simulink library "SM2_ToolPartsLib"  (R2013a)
settings: Solver=ode45  StartTime=0.0  StopTime=10.0  RelTol=1e-3
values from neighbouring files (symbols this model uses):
  m = v*BEAM.rho    [FlexBeamModelConstruct2.m]    (also in FlexBeamModelConstruct3.m = BEAM.rho*v; FlexBeam_1D_Construct.m = REF.m/REF.l*a.*(linspace(1-OPT.MassBiais+1e-6,1+OPT.MassBiai; FlexBeam_3D_Construct.m = REF.m/REF.l*a.*(linspace(1-OPT.MassBiais+1e-6,1+OPT.MassBiai; FreeFlexBeam_3D_Construct.m = REF.m/REF.l*a.*tmp2)
  N = D(1)+(H4^2+H3^2)/H2^2-(E(1)*H4+F(1)*H3)/H2    [MGD.m]    (also in MGD2.m)
  s = -sign(imag(KGZ_fr_tmp))    [LinprogReguliOptimFunc_1.m]    (also in LinprogReguliOptimFunc_2.m; LinprogReguliOptimFunc_1 - Copie.m)
  X = cos(phi(i))*x+sin(phi(i))*y    [MGI.m]
  Y = fft(y(:,i),NFFT)/L    [fft_bis.m]    (also in MGI.m = -sin(phi(i))*x+cos(phi(i))*y)
  Z = z    [MGI.m]
undefined symbols (not defined in the file or in its folder): deg, kg, SimParam
libraries: sm_lib x12, nesl_utility x1

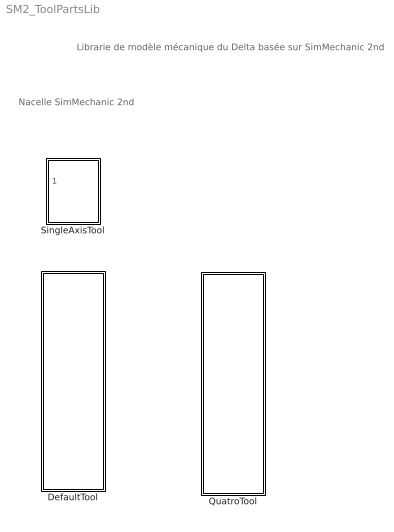
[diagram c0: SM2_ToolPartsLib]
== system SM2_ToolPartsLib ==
  note: Librarie de modèle mécanique du Delta basée sur SimMechanic 2nd
  note: Nacelle SimMechanic 2nd
  DefaultTool : Subsystem  InitFcn=SimParam.Tool = Tool_paramInitFnc(RawParam);
  QuatroTool : Subsystem  InitFcn=SimParam.Tool = Tool_paramInitFnc(RawParam);
  SingleAxisTool : Subsystem  InitFcn=SimParam.Tool = Tool_paramInitFnc(RawParam);

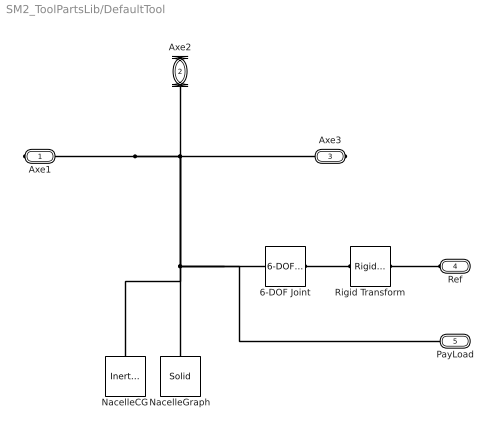
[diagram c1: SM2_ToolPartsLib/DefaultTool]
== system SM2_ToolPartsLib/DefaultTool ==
  6-DOF Joint : sm_lib/Joints/6-DOF Joint  SenseConstraintForceX=off  SenseConstraintForceY=off  SenseConstraintForceZ=off  SenseConstraintTorqueX=off  SenseConstraintTorqueY=off  SenseConstraintTorqueZ=off  ConstraintWrenchDir=FollowerOnBase  ConstraintWrenchFrame=BaseFrame  PxEquilibriumPosition=0  PxEquilibriumPositionUnits=m  PxSpringStiffness=0  PxSpringStiffnessUnits=N/m  PxDampingCoefficient=0  PxDampingCoefficientUnits=N/(m/s)  PxActuationMode=NoActuation  PxSensePosition=off  PxSenseVelocity=off  PxSenseAcceleration=off  PxSenseTorqueForce=off  PxPositionTargetValue=0  PxPositionTargetValueUnits=m  PxPositionTargetSpecify=on  PxPositionTargetPriority=Low  PxVelocityTargetValue=0  PxVelocityTargetValueUnits=m/s  PxVelocityTargetSpecify=on  PxVelocityTargetPriority=High  PyEquilibriumPosition=0  PyEquilibriumPositionUnits=m  PySpringStiffness=0  PySpringStiffnessUnits=N/m  PyDampingCoefficient=0  PyDampingCoefficientUnits=N/(m/s)  PyActuationMode=NoActuation  PySensePosition=off  PySenseVelocity=off  PySenseAcceleration=off  PySenseTorqueForce=off  PyPositionTargetValue=0  PyPositionTargetValueUnits=m  PyPositionTargetSpecify=on  PyPositionTargetPriority=Low  PyVelocityTargetValue=0  PyVelocityTargetValueUnits=m/s  PyVelocityTargetSpecify=on  PyVelocityTargetPriority=High  PzEquilibriumPosition=0  PzEquilibriumPositionUnits=m  PzSpringStiffness=0  PzSpringStiffnessUnits=N/m  PzDampingCoefficient=0  PzDampingCoefficientUnits=N/(m/s)  PzActuationMode=NoActuation  PzSensePosition=off  PzSenseVelocity=off  PzSenseAcceleration=off  PzSenseTorqueForce=off  PzPositionTargetValue=0  PzPositionTargetValueUnits=m  PzPositionTargetSpecify=on  PzPositionTargetPriority=Low  PzVelocityTargetValue=0  PzVelocityTargetValueUnits=m/s  PzVelocityTargetSpecify=on  PzVelocityTargetPriority=High  SphDefPosRotationMethod=None  SphDefPosRotationAngleUnits=deg  SphDefPosRotationStandardAxis=+Z  SphDefPosRotationAngle=0  SphDefPosRotationArbitraryAxis=[0 0 1]  SphDefPosFollAlignAxisA=+X  SphDefPosBaseAlignAxisA=+Y  SphDefPosFollAlignAxisB=+Y  SphDefPosBaseAlignAxisB=+Z  SphEqPosRotationMethod=None  SphEqPosRotationAngleUnits=deg  SphEqPosRotationStandardAxis=+Z  SphEqPosRotationAngle=0  SphEqPosRotationArbitraryAxis=[0 0 1]  SphEqPosFollAlignAxisA=+X  SphEqPosBaseAlignAxisA=+Y  SphEqPosFollAlignAxisB=+Y  SphEqPosBaseAlignAxisB=+Z  SphSpringStiffness=0  SphSpringStiffnessUnits=N*m/deg  SphDampingCoefficient=0  SphDampingCoefficientUnits=N*m/(deg/s)  SphActuateTorqueX=off  SphActuateTorqueY=off  SphActuateTorqueZ=off  SphActuateTorque=off  SphActuationMode=NoActuation  SphActuationFrame=BaseFrame  SphSensePosition=off  SphSenseVelocityX=off  SphSenseVelocityY=off  SphSenseVelocityZ=off  SphSenseVelocity=off  SphSenseAccelerationX=off  SphSenseAccelerationY=off  SphSenseAccelerationZ=off  SphSenseAcceleration=off  SphSenseTorqueX=off  SphSenseTorqueY=off  SphSenseTorqueZ=off  SphSenseTorqueForce=off  SphSensingFrame=BaseFrame  SphPositionTargetRotationMethod=AlignedAxes  SphPositionTargetRotationAngleUnits=deg  SphPositionTargetRotationStandardAxis=+Z  SphPositionTargetRotationAngle=0  SphPositionTargetRotationArbitraryAxis=[0 0 1]  SphPositionTargetFollAlignAxisA=+X  SphPositionTargetBaseAlignAxisA=+X  SphPositionTargetFollAlignAxisB=+Y  SphPositionTargetBaseAlignAxisB=+Y  SphPositionTargetSpecify=on  SphPositionTargetPriority=High  SphVelocityTargetValue=[0 0 0]  SphVelocityTargetValueUnits=deg/s  SphVelocityTargetSpecify=on  SphVelocityTargetPriority=High  SphVelocityTargetInFollowerFrame=on  BlockFunction=simmechanics.library.joints.sixdof_joint
  NacelleCG : sm_lib/Body Elements/Inertia  InertiaType=Custom  Mass=SimParam.Tool.m  MassUnits=kg  CenterOfMass=[0 0 0]  CenterOfMassUnits=m  MomentsOfInertia=SimParam.Tool.I'  MomentsOfInertiaUnits=kg*m^2  ProductsOfInertia=[0 0 0]  ProductsOfInertiaUnits=kg*m^2  BlockFunction=simmechanics.library.body_elements.inertia
  NacelleGraph : sm_lib/Body Elements/Solid  InertiaType=Custom  Mass=0  MassUnits=kg  CenterOfMass=[0 0 0]  CenterOfMassUnits=m  MomentsOfInertia=[0 0 0]  MomentsOfInertiaUnits=kg*m^2  ProductsOfInertia=[0 0 0]  ProductsOfInertiaUnits=kg*m^2  DensityBased=on  Density=1000  DensityUnits=kg/(m^3)  GraphicType=FromGeometry  MarkerShape=Sphere  MarkerSize=10  MarkerSizeUnits=m  GraphicVisPropType=SimpleVisualProperties  GraphicDiffuseColor=[0.5 0.5 0.5]  GraphicSpecularColor=[0.5 0.5 0.5 1.0]  GraphicAmbientColor=[0.15 0.15 0.15 1.0]  GraphicEmissiveColor=[0.0 0.0 0.0 1.0]  GraphicShininess=75  GraphicOpacity=1.0  GeometryShape=GeneralExtrusion  RectangleSize=[1 1]  RectangleSizeUnits=m  BrickDimensions=[1 1 1]  BrickDimensionUnits=m  CylinderRadius=1  CylinderRadiusUnits=m  CylinderLength=1  CylinderLengthUnits=m  SphereRadius=1  SphereRadiusUnits=m  EllipsoidRadii=[1 1 1]  EllipsoidRadiiUnits=m  ExtrusionCrossSection=1.5*SimParam.Tool.r.*[1 0;-0.5 0.866; -0.5 -0.866]  ExtrusionCrossSectionUnits=m  ExtrusionLength=0.01  ExtrusionLengthUnits=m  PolygonNumSides=3  PolygonOuterRadius=1  PolygonOuterRadiusUnits=m  ExtGeomFileUnits=m  RevolutionCrossSection=[1 1; 1 -1; 2 -1; 2 1]  RevolutionCrossSectionUnits=m  RevolutionExtent=Full  RevolutionAngle=180  RevolutionAngleUnits=deg  BlockFunction=simmechanics.library.body_elements.solid
  Rigid Transform : sm_lib/Frames and  Transforms/Rigid  Transform  TranslationMethod=Cartesian  TranslationLengthUnit=m  TranslationStandardAxis=+Z  TranslationStandardOffset=0  TranslationCartesianOffset=SimParam.IC.ToolPos0'  TranslationROffset=0  TranslationROffsetUnits=m  TranslationZOffset=0  TranslationZOffsetUnits=m  TranslationThetaOffset=0  TranslationThetaOffsetUnits=deg  RotationMethod=None  RotationAngleUnits=deg  RotationStandardAxis=+Z  RotationAngle=0  RotationArbitraryAxis=[0 0 1]  FollAlignAxisA=+X  BaseAlignAxisA=+Y  FollAlignAxisB=+Y  BaseAlignAxisB=+Z  BlockFunction=simmechanics.library.frames_transforms.rigid_transform
  Axe1 : PMIOPort  Port=1  Side=Right
  Axe2 : PMIOPort  Port=2  Side=Right
  Axe3 : PMIOPort  Port=3  Side=Right
  Ref : PMIOPort  Port=4  Side=Left
  PayLoad : PMIOPort  Port=5  Side=Left
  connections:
  Axe1/RConn1 -- 6-DOF Joint/RConn1 -- PayLoad/RConn1 -- NacelleGraph/RConn1 -- NacelleCG/RConn1 -- Axe2/RConn1 -- Axe3/RConn1
  Rigid Transform/RConn1 -- 6-DOF Joint/LConn1
  Rigid Transform/LConn1 -- Ref/RConn1

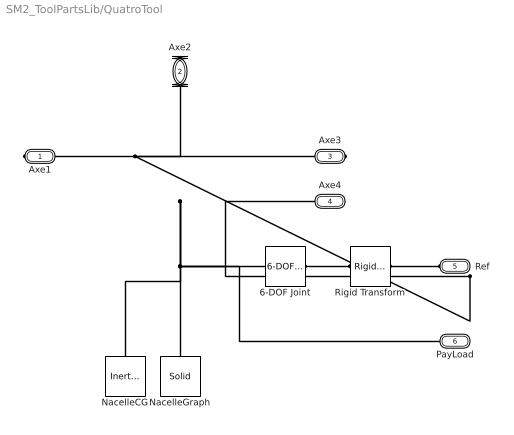
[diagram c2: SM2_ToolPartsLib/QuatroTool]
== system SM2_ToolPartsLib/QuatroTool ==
  6-DOF Joint : sm_lib/Joints/6-DOF Joint  SenseConstraintForceX=off  SenseConstraintForceY=off  SenseConstraintForceZ=off  SenseConstraintTorqueX=off  SenseConstraintTorqueY=off  SenseConstraintTorqueZ=off  ConstraintWrenchDir=FollowerOnBase  ConstraintWrenchFrame=BaseFrame  PxEquilibriumPosition=0  PxEquilibriumPositionUnits=m  PxSpringStiffness=0  PxSpringStiffnessUnits=N/m  PxDampingCoefficient=0  PxDampingCoefficientUnits=N/(m/s)  PxActuationMode=NoActuation  PxSensePosition=off  PxSenseVelocity=off  PxSenseAcceleration=off  PxSenseTorqueForce=off  PxPositionTargetValue=0  PxPositionTargetValueUnits=m  PxPositionTargetSpecify=on  PxPositionTargetPriority=Low  PxVelocityTargetValue=0  PxVelocityTargetValueUnits=m/s  PxVelocityTargetSpecify=on  PxVelocityTargetPriority=High  PyEquilibriumPosition=0  PyEquilibriumPositionUnits=m  PySpringStiffness=0  PySpringStiffnessUnits=N/m  PyDampingCoefficient=0  PyDampingCoefficientUnits=N/(m/s)  PyActuationMode=NoActuation  PySensePosition=off  PySenseVelocity=off  PySenseAcceleration=off  PySenseTorqueForce=off  PyPositionTargetValue=0  PyPositionTargetValueUnits=m  PyPositionTargetSpecify=on  PyPositionTargetPriority=Low  PyVelocityTargetValue=0  PyVelocityTargetValueUnits=m/s  PyVelocityTargetSpecify=on  PyVelocityTargetPriority=High  PzEquilibriumPosition=0  PzEquilibriumPositionUnits=m  PzSpringStiffness=0  PzSpringStiffnessUnits=N/m  PzDampingCoefficient=0  PzDampingCoefficientUnits=N/(m/s)  PzActuationMode=NoActuation  PzSensePosition=off  PzSenseVelocity=off  PzSenseAcceleration=off  PzSenseTorqueForce=off  PzPositionTargetValue=0  PzPositionTargetValueUnits=m  PzPositionTargetSpecify=on  PzPositionTargetPriority=Low  PzVelocityTargetValue=0  PzVelocityTargetValueUnits=m/s  PzVelocityTargetSpecify=on  PzVelocityTargetPriority=High  SphDefPosRotationMethod=None  SphDefPosRotationAngleUnits=deg  SphDefPosRotationStandardAxis=+Z  SphDefPosRotationAngle=0  SphDefPosRotationArbitraryAxis=[0 0 1]  SphDefPosFollAlignAxisA=+X  SphDefPosBaseAlignAxisA=+Y  SphDefPosFollAlignAxisB=+Y  SphDefPosBaseAlignAxisB=+Z  SphEqPosRotationMethod=None  SphEqPosRotationAngleUnits=deg  SphEqPosRotationStandardAxis=+Z  SphEqPosRotationAngle=0  SphEqPosRotationArbitraryAxis=[0 0 1]  SphEqPosFollAlignAxisA=+X  SphEqPosBaseAlignAxisA=+Y  SphEqPosFollAlignAxisB=+Y  SphEqPosBaseAlignAxisB=+Z  SphSpringStiffness=0  SphSpringStiffnessUnits=N*m/deg  SphDampingCoefficient=0  SphDampingCoefficientUnits=N*m/(deg/s)  SphActuateTorqueX=off  SphActuateTorqueY=off  SphActuateTorqueZ=off  SphActuateTorque=off  SphActuationMode=NoActuation  SphActuationFrame=BaseFrame  SphSensePosition=off  SphSenseVelocityX=off  SphSenseVelocityY=off  SphSenseVelocityZ=off  SphSenseVelocity=off  SphSenseAccelerationX=off  SphSenseAccelerationY=off  SphSenseAccelerationZ=off  SphSenseAcceleration=off  SphSenseTorqueX=off  SphSenseTorqueY=off  SphSenseTorqueZ=off  SphSenseTorqueForce=off  SphSensingFrame=BaseFrame  SphPositionTargetRotationMethod=AlignedAxes  SphPositionTargetRotationAngleUnits=deg  SphPositionTargetRotationStandardAxis=+Z  SphPositionTargetRotationAngle=0  SphPositionTargetRotationArbitraryAxis=[0 0 1]  SphPositionTargetFollAlignAxisA=+X  SphPositionTargetBaseAlignAxisA=+X  SphPositionTargetFollAlignAxisB=+Y  SphPositionTargetBaseAlignAxisB=+Y  SphPositionTargetSpecify=on  SphPositionTargetPriority=High  SphVelocityTargetValue=[0 0 0]  SphVelocityTargetValueUnits=deg/s  SphVelocityTargetSpecify=on  SphVelocityTargetPriority=High  SphVelocityTargetInFollowerFrame=on  BlockFunction=simmechanics.library.joints.sixdof_joint
  NacelleCG : sm_lib/Body Elements/Inertia  InertiaType=Custom  Mass=SimParam.Tool.m  MassUnits=kg  CenterOfMass=[0 0 0]  CenterOfMassUnits=m  MomentsOfInertia=SimParam.Tool.I'  MomentsOfInertiaUnits=kg*m^2  ProductsOfInertia=[0 0 0]  ProductsOfInertiaUnits=kg*m^2  BlockFunction=simmechanics.library.body_elements.inertia
  NacelleGraph : sm_lib/Body Elements/Solid  InertiaType=Custom  Mass=0  MassUnits=kg  CenterOfMass=[0 0 0]  CenterOfMassUnits=m  MomentsOfInertia=[0 0 0]  MomentsOfInertiaUnits=kg*m^2  ProductsOfInertia=[0 0 0]  ProductsOfInertiaUnits=kg*m^2  DensityBased=on  Density=1000  DensityUnits=kg/(m^3)  GraphicType=FromGeometry  MarkerShape=Sphere  MarkerSize=10  MarkerSizeUnits=m  GraphicVisPropType=SimpleVisualProperties  GraphicDiffuseColor=[0.5 0.5 0.5]  GraphicSpecularColor=[0.5 0.5 0.5 1.0]  GraphicAmbientColor=[0.15 0.15 0.15 1.0]  GraphicEmissiveColor=[0.0 0.0 0.0 1.0]  GraphicShininess=75  GraphicOpacity=1.0  GeometryShape=GeneralExtrusion  RectangleSize=[1 1]  RectangleSizeUnits=m  BrickDimensions=[1 1 1]  BrickDimensionUnits=m  CylinderRadius=1  CylinderRadiusUnits=m  CylinderLength=1  CylinderLengthUnits=m  SphereRadius=1  SphereRadiusUnits=m  EllipsoidRadii=[1 1 1]  EllipsoidRadiiUnits=m  ExtrusionCrossSection=1*SimParam.Tool.r.*[-1 1;-1 -1;1 -1;1 1]  ExtrusionCrossSectionUnits=m  ExtrusionLength=0.1*SimParam.Tool.r  ExtrusionLengthUnits=m  PolygonNumSides=3  PolygonOuterRadius=1  PolygonOuterRadiusUnits=m  ExtGeomFileUnits=m  RevolutionCrossSection=[1 1; 1 -1; 2 -1; 2 1]  RevolutionCrossSectionUnits=m  RevolutionExtent=Full  RevolutionAngle=180  RevolutionAngleUnits=deg  BlockFunction=simmechanics.library.body_elements.solid
  Rigid Transform : sm_lib/Frames and  Transforms/Rigid  Transform  TranslationMethod=Cartesian  TranslationLengthUnit=m  TranslationStandardAxis=+Z  TranslationStandardOffset=0  TranslationCartesianOffset=SimParam.IC.ToolPos0'  TranslationROffset=0  TranslationROffsetUnits=m  TranslationZOffset=0  TranslationZOffsetUnits=m  TranslationThetaOffset=0  TranslationThetaOffsetUnits=deg  RotationMethod=None  RotationAngleUnits=deg  RotationStandardAxis=+Z  RotationAngle=0  RotationArbitraryAxis=[0 0 1]  FollAlignAxisA=+X  BaseAlignAxisA=+Y  FollAlignAxisB=+Y  BaseAlignAxisB=+Z  BlockFunction=simmechanics.library.frames_transforms.rigid_transform
  Axe1 : PMIOPort  Port=1  Side=Right
  Axe2 : PMIOPort  Port=2  Side=Right
  Axe3 : PMIOPort  Port=3  Side=Right
  Axe4 : PMIOPort  Port=4  Side=Right
  Ref : PMIOPort  Port=5  Side=Left
  PayLoad : PMIOPort  Port=6  Side=Left
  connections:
  Axe1/RConn1 -- Axe4/RConn1 -- 6-DOF Joint/RConn1 -- PayLoad/RConn1 -- NacelleGraph/RConn1 -- NacelleCG/RConn1 -- Axe2/RConn1 -- Axe3/RConn1
  Rigid Transform/RConn1 -- 6-DOF Joint/LConn1
  Rigid Transform/LConn1 -- Ref/RConn1

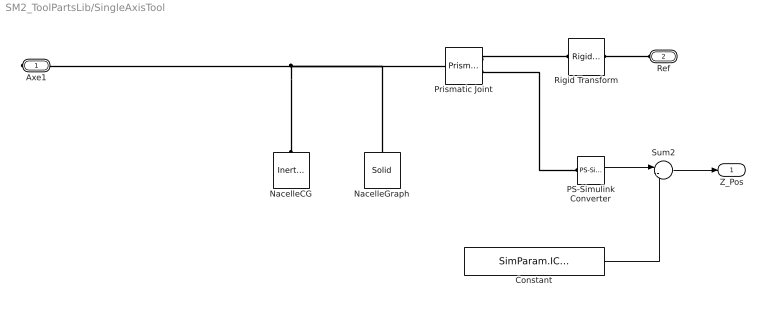
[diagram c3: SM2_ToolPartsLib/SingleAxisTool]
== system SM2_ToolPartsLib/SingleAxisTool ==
  Constant : Constant  Value=SimParam.IC.ToolPos0(3)
  NacelleCG : sm_lib/Body Elements/Inertia  InertiaType=Custom  Mass=SimParam.Tool.m  MassUnits=kg  CenterOfMass=[0 0 0]  CenterOfMassUnits=m  MomentsOfInertia=SimParam.Tool.I'  MomentsOfInertiaUnits=kg*m^2  ProductsOfInertia=[0 0 0]  ProductsOfInertiaUnits=kg*m^2  BlockFunction=simmechanics.library.body_elements.inertia
  NacelleGraph : sm_lib/Body Elements/Solid  InertiaType=Custom  Mass=0  MassUnits=kg  CenterOfMass=[0 0 0]  CenterOfMassUnits=m  MomentsOfInertia=[0 0 0]  MomentsOfInertiaUnits=kg*m^2  ProductsOfInertia=[0 0 0]  ProductsOfInertiaUnits=kg*m^2  DensityBased=on  Density=1000  DensityUnits=kg/(m^3)  GraphicType=FromGeometry  MarkerShape=Sphere  MarkerSize=10  MarkerSizeUnits=m  GraphicVisPropType=SimpleVisualProperties  GraphicDiffuseColor=[0.5 0.5 0.5]  GraphicSpecularColor=[0.5 0.5 0.5 1.0]  GraphicAmbientColor=[0.15 0.15 0.15 1.0]  GraphicEmissiveColor=[0.0 0.0 0.0 1.0]  GraphicShininess=75  GraphicOpacity=1.0  GeometryShape=GeneralExtrusion  RectangleSize=[1 1]  RectangleSizeUnits=m  BrickDimensions=[1 1 1]  BrickDimensionUnits=m  CylinderRadius=1  CylinderRadiusUnits=m  CylinderLength=1  CylinderLengthUnits=m  SphereRadius=1  SphereRadiusUnits=m  EllipsoidRadii=[1 1 1]  EllipsoidRadiiUnits=m  ExtrusionCrossSection=1.5*SimParam.Tool.r.*[1 0;-0.5 0.866; -0.5 -0.866]  ExtrusionCrossSectionUnits=m  ExtrusionLength=0.01  ExtrusionLengthUnits=m  PolygonNumSides=3  PolygonOuterRadius=1  PolygonOuterRadiusUnits=m  ExtGeomFileUnits=m  RevolutionCrossSection=[1 1; 1 -1; 2 -1; 2 1]  RevolutionCrossSectionUnits=m  RevolutionExtent=Full  RevolutionAngle=180  RevolutionAngleUnits=deg  BlockFunction=simmechanics.library.body_elements.solid
  PS-Simulink Converter : nesl_utility/PS-Simulink Converter  PhysicalDomain=network_engine_domain  SubClassName=ps_output  LeftPortType=input  RightPortType=output  PseudoPeriodic=off  Frequencies=[]  Unit=1  AffineConversion=off
  Prismatic Joint : sm_lib/Joints/Prismatic  Joint  SenseConstraintForceX=off  SenseConstraintForceY=off  SenseConstraintForceZ=off  SenseConstraintTorqueX=off  SenseConstraintTorqueY=off  SenseConstraintTorqueZ=off  ConstraintWrenchDir=FollowerOnBase  ConstraintWrenchFrame=BaseFrame  EquilibriumPosition=0  EquilibriumPositionUnits=m  SpringStiffness=0  SpringStiffnessUnits=N/m  DampingCoefficient=0  DampingCoefficientUnits=N/(m/s)  ActuationMode=NoActuation  SensePosition=on  SenseVelocity=off  SenseAcceleration=off  SenseTorqueForce=off  PositionTargetValue=0  PositionTargetValueUnits=m  PositionTargetSpecify=off  PositionTargetPriority=High  VelocityTargetValue=0  VelocityTargetValueUnits=m/s  VelocityTargetSpecify=off  VelocityTargetPriority=High  BlockFunction=simmechanics.library.joints.prismatic_joint
  Rigid Transform : sm_lib/Frames and  Transforms/Rigid  Transform  TranslationMethod=Cartesian  TranslationLengthUnit=m  TranslationStandardAxis=+Z  TranslationStandardOffset=0  TranslationCartesianOffset=SimParam.IC.ToolPos0'  TranslationROffset=0  TranslationROffsetUnits=m  TranslationZOffset=0  TranslationZOffsetUnits=m  TranslationThetaOffset=0  TranslationThetaOffsetUnits=deg  RotationMethod=None  RotationAngleUnits=deg  RotationStandardAxis=+Z  RotationAngle=0  RotationArbitraryAxis=[0 0 1]  FollAlignAxisA=+X  BaseAlignAxisA=+Y  FollAlignAxisB=+Y  BaseAlignAxisB=+Z  BlockFunction=simmechanics.library.frames_transforms.rigid_transform
  Sum2 : Sum  Inputs=|-+
  Axe1 : PMIOPort  Port=1  Side=Right
  Ref : PMIOPort  Port=2  Side=Left
  Z_Pos : Outport
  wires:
  PS-Simulink Converter/1 -> Sum2/1
  Sum2/1 -> Z_Pos/1
  Constant/1 -> Sum2/2
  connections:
  NacelleCG/RConn1 -- Prismatic Joint/LConn1 -- NacelleGraph/RConn1 -- Axe1/RConn1
  Prismatic Joint/RConn1 -- Rigid Transform/RConn1
  Rigid Transform/LConn1 -- Ref/RConn1
  PS-Simulink Converter/LConn1 -- Prismatic Joint/RConn2
